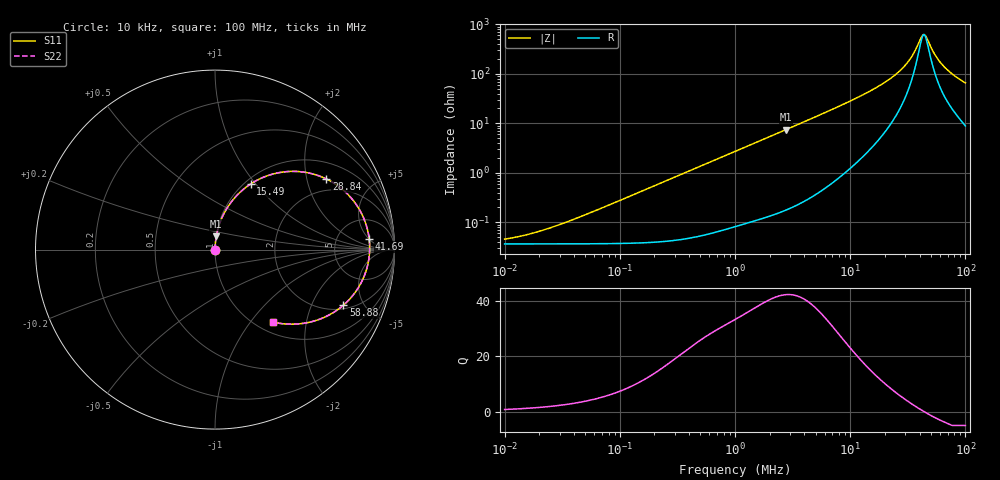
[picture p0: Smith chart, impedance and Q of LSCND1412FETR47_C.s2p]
! LSCND1412FETR47_C  S-PARAMETER MODEL  ( Standard Model )
! Model Generated by TAIYO YUDEN Corporation (http://www.ty-top.com)
! Version 1.0
! TAIYO YUDEN Control No. 201211
! Copyright(c) 2020 TAIYO YUDEN CO.,LTD. All Rights Reserved.
! Product Description (link to TY-COMPAS)
! https://ds.yuden.co.jp/TYCOMPAS/or/detail?pn=LSCND1412FETR47MC&u=M
! Products Name : Inductors
! Characteristics :
!  Inductance : 0.47 [uH] , SRF(min) : - [Hz] , DC Resistance(max) : 42 [mOhm]
!  Rated Current : Saturation  3.0 [A] (dL = 30 [%]), Temp Rise  3.1 [A] (dT = 40 [degC])
!  Case Size : 1.4 x 1.2 / 0.055 x 0.047 [mm/inch] , Thickness : 0.65 / 0.026 [mm/inch]
!  (Conditions: Temperature = 25 [degC] , DC Bias Current = 0 [A])
! External Node Assignments :
!  1  o---GGG---o  2
! GND o---------o GND
! Frequency Range : 10kHz  -  100MHz  [ 402 STEP ]
# MHz S RI R 50
! Freq[MHz].  S11 Real  S11 Imag  S21 Real  S21 Imag  S12 Real  S12 Imag  S22 Real  S22 Imag
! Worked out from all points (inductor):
!   401 points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, 10 kHz to 100 MHz, reference 50 ohm
!   read as one part in series: L = 436 nH near 40.74 kHz
!   highest Q = 42.1 at 2.754 MHz (marker M1), where L = 428 nH
!   self-resonance near 43.71 MHz
!   S11 on the Smith chart (normalised r, x): 10 kHz: 1.00, +0.00; 15.49 MHz: 1.07, +0.94; 28.84 MHz: 1.54, +2.63; 41.69 MHz: 11, +5; 58.88 MHz: 2.22, -3.50; 100 MHz: 1.18, -1.30
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0.01  0.000367 0.000274  0.9996 -0.000274  0.9996 -0.000274  0.000367 0.000274
0.019953  0.000367 0.000547  0.9996 -0.000547  0.9996 -0.000547  0.000367 0.000547
0.046774  0.00037 0.00128  0.9996 -0.00128  0.9996 -0.00128  0.00037 0.00128
0.218776  0.000439 0.00599  0.9996 -0.00599  0.9996 -0.00599  0.000439 0.00599
1  0.00155 0.027  0.9985 -0.027  0.9985 -0.027  0.00155 0.027
2.754229  0.00719 0.0735  0.9928 -0.0735  0.9928 -0.0735  0.00719 0.0735
4.677351  0.0189 0.1238  0.9811 -0.1238  0.9811 -0.1238  0.0189 0.1238
9.549926  0.0759 0.2447  0.9241 -0.2447  0.9241 -0.2447  0.0759 0.2447
15.48817  0.1989 0.3658  0.8011 -0.3658  0.8011 -0.3658  0.1989 0.3658
21.87762  0.3886 0.4334  0.6114 -0.4334  0.6114 -0.4334  0.3886 0.4334
25.11886  0.4975 0.4313  0.5025 -0.4313  0.5025 -0.4313  0.4975 0.4313
28.84032  0.62 0.3938  0.38 -0.3938  0.38 -0.3938  0.62 0.3938
31.62278  0.7019 0.3424  0.2981 -0.3424  0.2981 -0.3424  0.7019 0.3424
34.67368  0.7751 0.2675  0.2249 -0.2675  0.2249 -0.2675  0.7751 0.2675
41.68694  0.8591 0.0595  0.1409 -0.0595  0.1409 -0.0595  0.8591 0.0595
43.65158  0.8618 0.00144  0.1382 -0.00144  0.1382 -0.00144  0.8618 0.00144
45.70882  0.8566 -0.0562  0.1434 0.0562  0.1434 0.0562  0.8566 -0.0562
52.48075  0.7985 -0.2124  0.2015 0.2124  0.2015 0.2124  0.7985 -0.2124
58.88437  0.7155 -0.3097  0.2845 0.3097  0.2845 0.3097  0.7155 -0.3097
66.06934  0.62 -0.3723  0.38 0.3723  0.38 0.3723  0.62 -0.3723
74.13102  0.5254 -0.4049  0.4746 0.4049  0.4746 0.4049  0.5254 -0.4049
100  0.3226 -0.4042  0.6774 0.4042  0.6774 0.4042  0.3226 -0.4042
